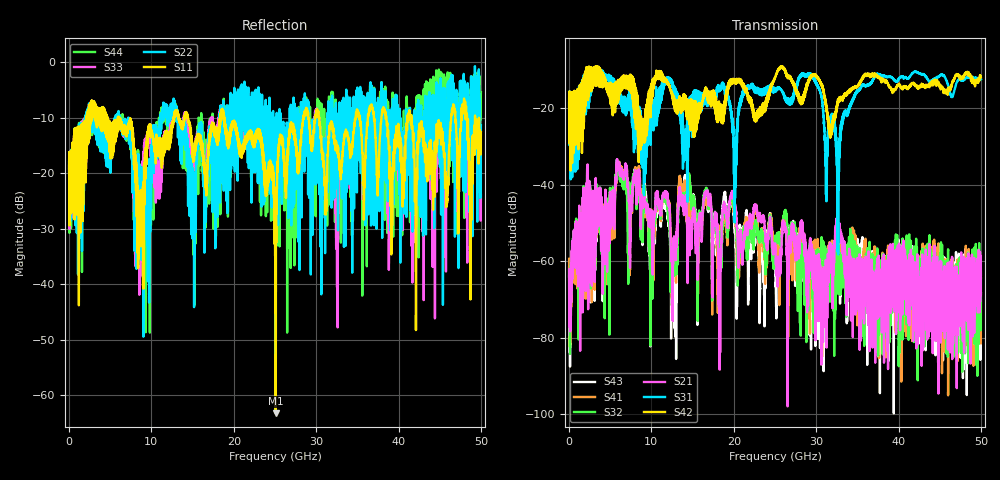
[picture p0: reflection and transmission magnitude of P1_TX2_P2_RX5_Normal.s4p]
!Keysight Technologies,N5225B,MY57041031,A.13.20.10
!Date: Friday, May 31, 2019 11:35:06
!Correction: S11(Full 4 Port(1,2,3,4))
!S12(Full 4 Port(1,2,3,4))
!S13(Full 4 Port(1,2,3,4))
!S14(Full 4 Port(1,2,3,4))
!S21(Full 4 Port(1,2,3,4))
!S22(Full 4 Port(1,2,3,4))
!S23(Full 4 Port(1,2,3,4))
!S24(Full 4 Port(1,2,3,4))
!S31(Full 4 Port(1,2,3,4))
!S32(Full 4 Port(1,2,3,4))
!S33(Full 4 Port(1,2,3,4))
!S34(Full 4 Port(1,2,3,4))
!S41(Full 4 Port(1,2,3,4))
!S42(Full 4 Port(1,2,3,4))
!S43(Full 4 Port(1,2,3,4))
!S44(Full 4 Port(1,2,3,4))
!S4P File: Measurements: <S11,S12,S13,S14>,
!<S21,S22,S23,S24>,
!<S31,S32,S33,S34>,
!<S41,S42,S43,S44>:
# Hz S  dB  R 50.0
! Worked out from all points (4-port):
!   5000 points, 10 MHz to 50 GHz, reference 50 ohm
!   strongest paths, dB at 10 MHz, 12.51 GHz, 25.01 GHz, 37.51 GHz, 50 GHz:
!     S42: -19.4, -17.0, -11.9, -11.9, -12.0
!     S31: -19.5, -13.0, -15.4, -11.2, -12.5
!     S21: -64.0, -62.0, -56.5, -64.0, -63.6
!     S32: -62.4, -66.2, -55.2, -67.6, -64.3
!     S41: -59.3, -73.3, -55.4, -71.0, -70.3
!     S43: -61.7, -60.6, -59.9, -61.0, -68.4
!   lowest |S11| = -63.2 dB at 25.1 GHz (marker M1), VSWR 1.00, Z = 49.9 + j0.033 ohm
!   |S11| at or under -10 dB: 6.091 GHz to 12.71 GHz (6.616 GHz wide, 70.4 % of centre); 18.82 GHz to 28.43 GHz (9.605 GHz wide, 40.7 % of centre); 41.57 GHz to 46.38 GHz (4.809 GHz wide, 10.9 % of centre)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
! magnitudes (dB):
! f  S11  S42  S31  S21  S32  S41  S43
! 10 MHz  -19.7  -19.4  -19.5  -64.0  -62.4  -59.3  -61.7
! 5.99 GHz  -10.5  -17.1  -16.0  -35.0  -35.6  -35.2  -35.8
! 12.8 GHz  -9.3  -19.8  -14.6  -54.5  -58.5  -56.8  -63.0
! 14.34 GHz  -9.3  -20.4  -29.3  -51.4  -43.6  -48.2  -37.7
! 25.1 GHz  -63.2  -11.5  -15.1  -59.4  -55.3  -56.1  -66.0
! 32.64 GHz  -15.8  -18.3  -37.5  -50.8  -66.1  -53.4  -57.7
! 50 GHz  -12.6  -12.0  -12.5  -63.6  -64.3  -70.3  -68.4
